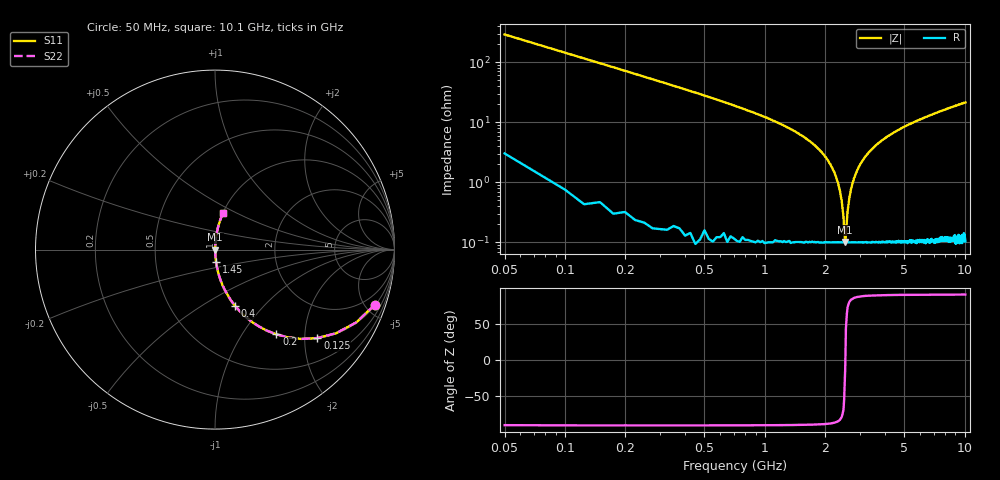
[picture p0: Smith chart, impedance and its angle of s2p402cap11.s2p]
! AVX Thin Film Operation		Date: April 2003
! Description: Accu-P® Series, Thin Film, SMD, RF Capacitor
! Part Number: 04023J110FBS
! 50 MHz  -  10.05 GHz
! Serial Measurements
# hz S db R 50
!	S11		S21		S12		S22
!	dB	Phase	dB	Phase	dB	Phase	dB	Phase
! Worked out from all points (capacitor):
!   400 points, 50 MHz to 10.1 GHz, reference 50 ohm
!   read as one part in series: C = 11 pF near 100 MHz
!   lowest |Z| = 101 mohm at 2.53 GHz (marker M1)
!   series resonance near 2.533 GHz, so ESL is about 360 pH
!   S11 on the Smith chart (normalised r, x): 50 MHz: 1.06, -5.79; 125 MHz: 1.01, -2.31; 200 MHz: 1.01, -1.44; 400 MHz: 1.00, -0.71; 1.45 GHz: 1.00, -0.13; 10.1 GHz: 1.00, +0.43
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5e7  -0.52 -19.0  -9.74 70.4  -9.74 70.4  -0.52 -19.0
1.25e8  -2.45 -40.8  -3.70 49.0  -3.70 49.0  -2.45 -40.8
2e8  -4.69 -54.1  -1.82 35.6  -1.82 35.6  -4.69 -54.1
4e8  -9.57 -70.4  -0.52 19.4  -0.52 19.4  -9.57 -70.4
7.75e8  -15.60 -80.0  -0.13 9.6  -0.13 9.6  -15.60 -80.0
1.45e9  -23.50 -85.3  -0.03 3.8  -0.03 3.8  -23.50 -85.3
1.73e9  -27.00 -86.1  -0.02 2.6  -0.02 2.6  -27.00 -86.1
2.08e9  -32.80 -86.2  -0.01 1.3  -0.01 1.3  -32.80 -86.2
2.33e9  -40.30 -83.5  -0.01 0.6  -0.01 0.6  -40.30 -83.5
2.43e9  -46.20 -78.0  -0.01 0.3  -0.01 0.3  -46.20 -78.0
2.48e9  -51.50 -67.9  -0.01 0.1  -0.01 0.1  -51.50 -67.9
2.53e9  -59.90 -10.6  -0.01 0.0  -0.01 0.0  -59.90 -10.6
2.6e9  -49.60 72.3  -0.01 -0.2  -0.01 -0.2  -49.60 72.3
2.65e9  -45.30 79.1  -0.01 -0.3  -0.01 -0.3  -45.30 79.1
2.75e9  -40.30 83.5  -0.01 -0.5  -0.01 -0.5  -40.30 83.5
3e9  -34.10 86.0  -0.01 -1.1  -0.01 -1.1  -34.10 86.0
3.4e9  -29.30 86.4  -0.01 -2.0  -0.01 -2.0  -29.30 86.4
4.1e9  -24.80 85.7  -0.02 -3.3  -0.02 -3.3  -24.80 85.7
5.08e9  -21.30 84.4  -0.04 -4.9  -0.04 -4.9  -21.30 84.4
6.75e9  -17.70 82.1  -0.08 -7.5  -0.08 -7.5  -17.70 82.1
8.43e9  -15.40 79.8  -0.14 -9.8  -0.14 -9.8  -15.40 79.8
1.01e10  -13.60 77.7  -0.20 -12.0  -0.20 -12.0  -13.60 77.7
